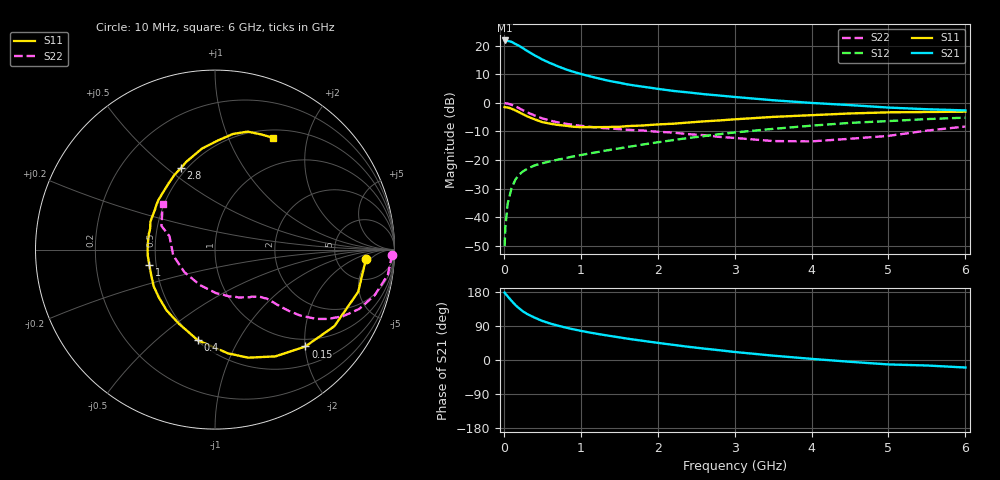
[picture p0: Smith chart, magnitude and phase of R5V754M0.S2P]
! SIEMENS Small Signal Semiconductors
! BFR183
! Si NPN RF Bipolar Junction Transistor in SOT23
! VCE = 0.75 V  IC = 4 mA
! Common Emitter S-Parameters:  May  1996
# GHz  S  MA  R  50
!  f  S11  S21  S12  S22
! GHz  MAG  ANG  MAG  ANG  MAG  ANG  MAG  ANG
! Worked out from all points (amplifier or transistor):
!   36 points, 10 MHz to 6 GHz, reference 50 ohm
!   highest |S21| = 21.8 dB at 10 MHz (marker M1)
!   |S21| within 3 dB of that: start of sweep to 265.4 MHz
!   unconditionally stable (mu >= 1): 1.057 GHz to 3.044 GHz
!   at 250 MHz: K = 0.37, MSG = 21.5 dB, |S12| = -24.0 dB
!   at 1.4 GHz: K = 1.09, MAG = 10.2 dB, |S12| = -16.4 dB
!   at 6 GHz: K = 0.95, MSG = 1.3 dB, |S12| = -5.2 dB
!   S11 on the Smith chart (normalised r, x): 10 MHz: 10, -4; 150 MHz: 0.85, -2.01; 400 MHz: 0.51, -0.70; 1 GHz: 0.46, -0.09; 2.8 GHz: 0.47, +0.56; 6 GHz: 0.60, +1.47
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0.01  0.842 -3.5  12.36 177.8  0.0031 90.1  0.9885 -1.6
0.02  0.836 -6.8  12.18 175.0  0.0067 83.8  0.9821 -3.4
0.05  0.8319 -16.4  12.12 167.8  0.0173 81.6  0.9731 -8.3
0.1  0.7902 -32.7  11.71 156.1  0.0322 73.4  0.9252 -16.0
0.15  0.7379 -47.0  10.73 145.1  0.0453 66.2  0.8685 -22.4
0.2  0.6835 -60.5  9.939 136.1  0.0556 61.6  0.8052 -27.4
0.25  0.63 -72.9  9.034 128.0  0.0633 56.8  0.7394 -31.5
0.3  0.5829 -82.8  8.145 121.8  0.0696 54.1  0.6857 -34.3
0.4  0.5144 -100.6  6.799 111.8  0.0804 50.4  0.6013 -37.7
0.5  0.4595 -115.9  5.743 103.1  0.0876 48.6  0.5351 -39.7
0.6  0.4326 -128.7  4.979 96.4  0.0947 48.1  0.4891 -40.9
0.8  0.3982 -149.1  3.88 85.8  0.108 48.2  0.4313 -42.3
1  0.3753 -167.2  3.207 77.0  0.1219 49.3  0.3965 -43.5
1.1  0.3764 -174.9  2.961 73.1  0.1291 49.8  0.383 -44.7
1.3  0.3762 172.3  2.546 66.1  0.1442 50.5  0.3614 -46.6
1.6  0.3916 156.8  2.112 56.5  0.1682 50.8  0.3382 -50.9
2.2  0.4314 131.9  1.619 40.0  0.2227 49.2  0.3017 -62.6
2.8  0.492 112.7  1.344 25.8  0.2826 44.8  0.2538 -80.4
3.5  0.5674 97.4  1.111 11.5  0.3504 37.0  0.2144 -113.2
4.5  0.652 81.2  0.913 -4.7  0.4464 24.4  0.2351 -171.9
5.5  0.6914 68.2  0.773 -14.5  0.5197 12.2  0.3266 156.1
6  0.7012 62.8  0.737 -19.8  0.5508 4.2  0.3851 139.1
